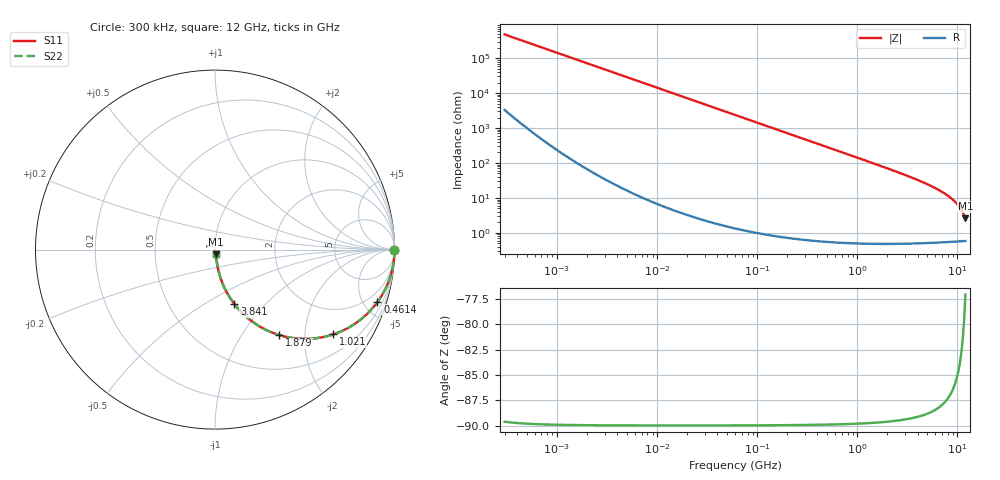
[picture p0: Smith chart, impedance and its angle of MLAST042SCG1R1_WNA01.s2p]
! MLAST042SCG1R1_WNA01  S-PARAMETER MODEL  ( General Type )
! Model Generated by TAIYO YUDEN Corporation (http://www.ty-top.com)
! Version 1.0
! TAIYO YUDEN Control No. 150820
! Copyright(c) 2015 TAIYO YUDEN CO.,LTD. All Rights Reserved.
! Product Description (link to TY-COMPAS)
! https://ds.yuden.co.jp/TYCOMPAS/or/detail?pn=MLAST042SCG1R1AWNA01&u=M
! Products Name : Multilayer Ceramic Capacitors
! Characteristics :
!  Capacitance : 1.1 pF , Rated Voltage : 25V , TCC : CG / C0G
!  Case Size : 0.4 x 0.2 / 0.016 x 0.008 [mm/inch] , Thickness : 0.2 / 0.008 [mm/inch]
!  (Conditions: Temperature = 25 degC , DC Bias Current/Voltage = 0A / 0V)
! External Node Assignments :
!  1  o---| |---o  2
! GND o---------o GND
! Frequency Range : 0.3MHz  -  12000MHz  [ 401 STEP ]
# MHz S RI R 50
! Freq[MHz].  S11 Real  S11 Imag  S21 Real  S21 Imag  S12 Real  S12 Imag  S22 Real  S22 Imag
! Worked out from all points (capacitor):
!   401 points, 300 kHz to 12 GHz, reference 50 ohm
!   read as one part in series: C = 1.11 pF near 316.3 kHz
!   lowest |Z| = 2.61 ohm at 12 GHz (marker M1)
!   S11 on the Smith chart (normalised r, x): 300 kHz: open; 461.4 MHz: 1.01, -6.19; 1.021 GHz: 1.01, -2.78; 1.879 GHz: 1.01, -1.49; 3.841 GHz: 1.01, -0.68; 12 GHz: 1.01, -0.05
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0.3  1 -0.00021  1.49e-06 0.00021  1.49e-06 0.00021  1 -0.00021
1.769972  1 -0.00124  2.78e-06 0.00124  2.78e-06 0.00124  1 -0.00124
10.44266  0.9999 -0.0073  5.67e-05 0.0073  5.67e-05 0.0073  0.9999 -0.0073
60  0.9982 -0.0419  0.00178 0.0419  0.00178 0.0419  0.9982 -0.0419
159.8975  0.9876 -0.1104  0.0124 0.1104  0.0124 0.1104  0.9876 -0.1104
353.9943  0.9419 -0.2332  0.0581 0.2332  0.0581 0.2332  0.9419 -0.2332
461.3684  0.9051 -0.2921  0.0949 0.2921  0.0949 0.2921  0.9051 -0.2921
686.4755  0.8114 -0.3899  0.1886 0.3899  0.1886 0.3899  0.8114 -0.3899
1021.415  0.6592 -0.4722  0.3408 0.4722  0.3408 0.4722  0.6592 -0.4722
1403.667  0.504 -0.4976  0.496 0.4976  0.496 0.4976  0.504 -0.4976
1878.541  0.3589 -0.4765  0.6411 0.4765  0.6411 0.4765  0.3589 -0.4765
2088.533  0.3102 -0.459  0.6898 0.459  0.6898 0.459  0.3102 -0.459
2795.104  0.196 -0.392  0.804 0.392  0.804 0.392  0.196 -0.392
3841.137  0.1084 -0.3038  0.8916 0.3038  0.8916 0.3038  0.1084 -0.3038
5868.704  0.0423 -0.1885  0.9577 0.1885  0.9577 0.1885  0.0423 -0.1885
7064.448  0.0262 -0.1427  0.9738 0.1427  0.9738 0.1427  0.0262 -0.1427
8064.993  0.0181 -0.1117  0.9819 0.1117  0.9819 0.1117  0.0181 -0.1117
8966.534  0.0133 -0.0878  0.9867 0.0878  0.9867 0.0878  0.0133 -0.0878
9968.853  0.00983 -0.0646  0.9902 0.0646  0.9902 0.0646  0.00983 -0.0646
10793.46  0.00798 -0.0475  0.992 0.0475  0.992 0.0475  0.00798 -0.0475
11380.75  0.00708 -0.0363  0.9929 0.0363  0.9929 0.0363  0.00708 -0.0363
12000  0.00645 -0.0251  0.9936 0.0251  0.9936 0.0251  0.00645 -0.0251
